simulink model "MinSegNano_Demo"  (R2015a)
settings: Solver=ode45  StartTime=0.0  StopTime=10.0  RelTol=1e-3
libraries: RASPlib x10, arduinolib x4, MinSegLibrary_MinSegNano x2

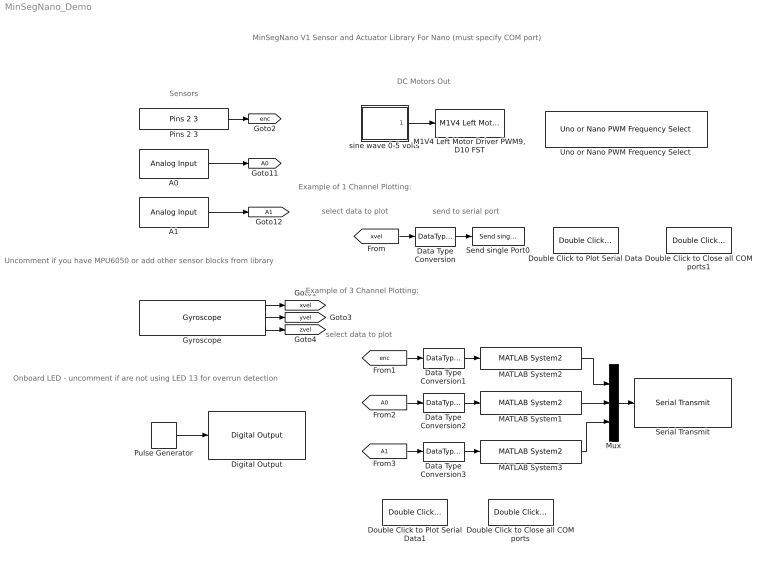
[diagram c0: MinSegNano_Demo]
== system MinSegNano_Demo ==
  note: Onboard LED - uncomment if are not using LED 13 for overrun detection
  note: Uncomment if you have MPU6050 or add other sensor blocks from library
  note: Example of 1 Channel Plotting:
  note: send to serial port
  note: select data to plot
  note: DC Motors Out
  note: Sensors
  note: MinSegNano V1 Sensor and Actuator Library For Nano (must specify COM port)
  note: Example of 3 Channel Plotting:
  note: select data to plot
  A0 : arduinolib/Analog Input  pinNumber=0  sampleTime=-1  blockPlatform=arduino
  A1 : arduinolib/Analog Input  pinNumber=1  sampleTime=-1  blockPlatform=arduino
  Data Type Conversion : DataTypeConversion  Commented=on  OutDataTypeStr=single
  Data Type Conversion1 : DataTypeConversion  OutDataTypeStr=single
  Data Type Conversion2 : DataTypeConversion  OutDataTypeStr=single
  Data Type Conversion3 : DataTypeConversion  OutDataTypeStr=single
  Digital Output : arduinolib/Digital Output  Commented=on  pinNumber=13  blockPlatform=arduino
  Double Click to Close all COM ports : RASPlib/Double Click to Close all COM ports
  Double Click to Close all COM ports1 : RASPlib/Double Click to Close all COM ports  Commented=on
  Double Click to Plot Serial Data : RASPlib/Double Click to Plot Serial Data  Commented=on  COMport=5  BaudRate=9600  NumSamples=500  DataType=single  Ncx=1
  Double Click to Plot Serial Data1 : RASPlib/Double Click to Plot Serial Data  COMport=5  BaudRate=9600  NumSamples=500  DataType=single  Ncx=3
  Gyroscope : RASPlib/Gyroscope  Commented=on  DLPFmode=0
  "M1V4 Left Motor Driver PWM9, D10 FST" : MinSegLibrary_MinSegNano/M1V4 Left Motor Driver PWM9, D10 FST  Vsupply=3.25
  MATLAB System1 : RASPlib/Send single Port0/MATLAB System2  SimulateUsing=Code generation
  MATLAB System2 : RASPlib/Send single Port0/MATLAB System2  SimulateUsing=Code generation
  MATLAB System3 : RASPlib/Send single Port0/MATLAB System2  SimulateUsing=Code generation
  Mux : Mux  Inputs=3
  Pins 2 3 : MinSegLibrary_MinSegNano/Pins 2 3  Encoder=0  PinA=2  PinB=3
  Pulse Generator : DiscretePulseGenerator  Commented=on  PulseType=Time based  Period=10  PulseWidth=5
  Send single Port0 : RASPlib/Send single Port0  Commented=on
  Serial Transmit : arduinolib/Serial Transmit  portNumber=0  blockPlatform=arduino
  Uno or Nano PWM Frequency Select : RASPlib/Uno or Nano PWM Frequency Select  Frequency=490Hz  Timer=1 - pins 9, 10
  sine wave 0-5 volts : Subsystem
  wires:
  sine wave 0-5 volts/1(sine) -> "M1V4 Left Motor Driver PWM9, D10 FST"/1
  A0/1 -> [A0]
  A1/1 -> [A1]
  Pins 2 3/1 -> [enc]
  [xvel] -> Data Type Conversion/1
  Data Type Conversion/1 -> Send single Port0/1
  Gyroscope/1 -> [xvel]
  MATLAB System1/1 -> Mux/2
  MATLAB System2/1 -> Mux/1
  [enc] -> Data Type Conversion1/1
  Data Type Conversion1/1 -> MATLAB System2/1
  [A0] -> Data Type Conversion2/1
  Data Type Conversion2/1 -> MATLAB System1/1
  Mux/1 -> Serial Transmit/1
  Data Type Conversion3/1 -> MATLAB System3/1
  MATLAB System3/1 -> Mux/3
  [A1] -> Data Type Conversion3/1
  Pulse Generator/1 -> Digital Output/1
  Gyroscope/2 -> [yvel]
  Gyroscope/3 -> [zvel]

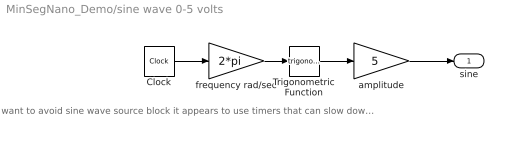
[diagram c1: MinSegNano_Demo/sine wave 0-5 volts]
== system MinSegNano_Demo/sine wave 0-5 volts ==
  note: want to avoid sine wave source block it appears to use timers that can slow down the serial port data transimission, and maybe other timers use a clock instead like this
  Clock : Clock
  Trigonometric Function : Trigonometry
  amplitude : Gain  Gain=5
  frequency rad/sec : Gain  Gain=2*pi
  sine : Outport
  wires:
  Clock/1 -> frequency rad/sec/1
  Trigonometric Function/1 -> amplitude/1
  frequency rad/sec/1 -> Trigonometric Function/1
  amplitude/1 -> sine/1
